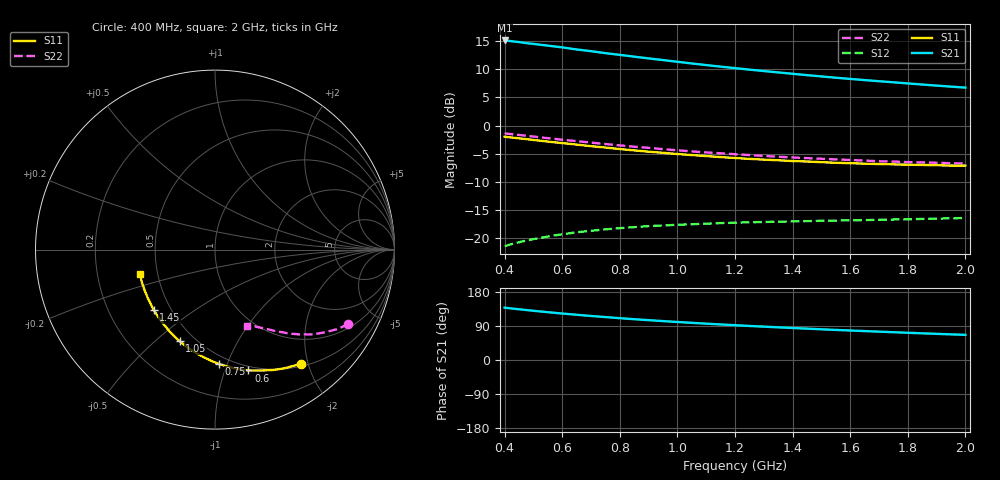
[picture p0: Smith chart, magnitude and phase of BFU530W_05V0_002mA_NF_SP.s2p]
! Filename:  P:\Prog\Test\Noise\ATS_data\Testdata_Net\06 Compressed Noise after Statistics\BFU530W_APM2013_09_A05_05p0V_002mA_NF_CM01_D.sf
! Date/Time: Tue 26/Mar/2013 18:06:06
! BFU530W_APM2013_09_A05_05p0V_1to25mA_NF_CM01_Bias2_R.sf
! Noise Parameter Data File
! BFU530W_APM2013_09_A05_05p0V_1to25mA_NF_CM01
! Date/time: Thu Mar 21 20:31:54 2013
! VAR V_out= 5.001000
! VAR I_out= 2.005000
! VAR V_in= 0.798700
! VAR I_in= 0.020605
! Device data file deembeded for feedlines and parallel
! Original file: \06 Compressed Noise after Statistics\BFU530W_APM2013_09_A05_05p0V_002mA_NF_CM01_R.sf
! Feed-files: PR019V01_070313_Feed1.s2p, PR019V01_070313_Feed2.s2p
! Parallel-file: PR019V01_070313_Par.s2p
# MHz S MA R 50
!  Freq-MHz  S11-mag  S11-arg  S21-mag  S21-arg  S12-mag  S12-arg  S22-mag  S22-arg
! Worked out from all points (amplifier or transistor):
!   37 points, 400 MHz to 2 GHz, reference 50 ohm
!   highest |S21| = 15.1 dB at 400 MHz (marker M1)
!   |S21| within 3 dB of that: start of sweep to 870.1 MHz
!   unconditionally stable (mu >= 1): nowhere
!   at 500 MHz: K = 0.28, MSG = 17.3 dB, |S12| = -20.2 dB
!   at 1.1 GHz: K = 0.58, MSG = 14.1 dB, |S12| = -17.4 dB
!   at 2 GHz: K = 0.95, MSG = 11.6 dB, |S12| = -16.4 dB
!   lowest NFmin = 0.49 dB at 420 MHz
!   S11 on the Smith chart (normalised r, x): 400 MHz: 0.54, -1.88; 600 MHz: 0.46, -1.21; 750 MHz: 0.44, -0.93; 1.05 GHz: 0.41, -0.60; 1.45 GHz: 0.40, -0.35; 2 GHz: 0.40, -0.14
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400  0.7951 -53.0  5.685 138.1  0.08496 60.0  0.8499 -29.1
420  0.7841 -55.4  5.618 136.3  0.08795 58.9  0.8397 -30.2
440  0.7745 -57.6  5.537 134.7  0.09071 57.8  0.8295 -31.3
480  0.7549 -62.0  5.363 131.5  0.09582 55.8  0.8089 -33.3
500  0.7445 -64.3  5.299 129.9  0.09817 54.8  0.7979 -34.2
550  0.72 -69.4  5.115 126.2  0.1035 52.7  0.7721 -36.5
600  0.6982 -74.6  4.935 122.6  0.1084 50.7  0.7479 -38.5
650  0.6773 -79.1  4.729 119.4  0.1128 48.9  0.727 -40.3
700  0.6555 -83.9  4.569 116.1  0.1163 47.3  0.7047 -42.2
750  0.6376 -88.1  4.385 113.2  0.1198 45.9  0.6846 -43.6
850  0.6013 -96.5  4.082 107.6  0.1254 43.5  0.6483 -46.5
950  0.5721 -104.1  3.808 102.7  0.1296 41.6  0.6168 -49.1
1050  0.5467 -111.2  3.552 98.1  0.133 40.3  0.589 -51.2
1150  0.5247 -118.0  3.329 93.8  0.1362 39.1  0.5671 -53.2
1200  0.5148 -121.0  3.231 91.8  0.1371 38.8  0.5562 -54.2
1300  0.498 -127.2  3.043 88.0  0.1392 38.2  0.537 -56.0
1450  0.4793 -135.6  2.799 82.7  0.1418 38.0  0.5135 -58.5
1500  0.4728 -138.3  2.725 81.0  0.1427 38.0  0.507 -59.4
1600  0.4632 -143.5  2.591 77.8  0.144 38.3  0.4945 -61.0
1750  0.4521 -150.7  2.417 73.3  0.1465 39.1  0.4785 -63.3
1850  0.4469 -155.3  2.31 70.4  0.1483 39.7  0.4706 -64.8
2000  0.441 -161.9  2.169 66.3  0.1512 41.1  0.46 -67.2
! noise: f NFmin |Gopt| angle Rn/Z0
400  0.4932  0.4795  26.13  0.1822
460  0.507  0.4748  29.77  0.1833
600  0.554  0.4657  38.18  0.1855
800  0.6099  0.4669  51.35  0.1631
1000  0.663  0.4618  64.64  0.1645
1200  0.7036  0.4446  78.13  0.1471
1400  0.7768  0.4414  90.96  0.1221
1600  0.6909  0.4512  106.1  0.1007
1800  0.845  0.4085  118.2  0.098
2000  0.9167  0.4056  131.3  0.0905
